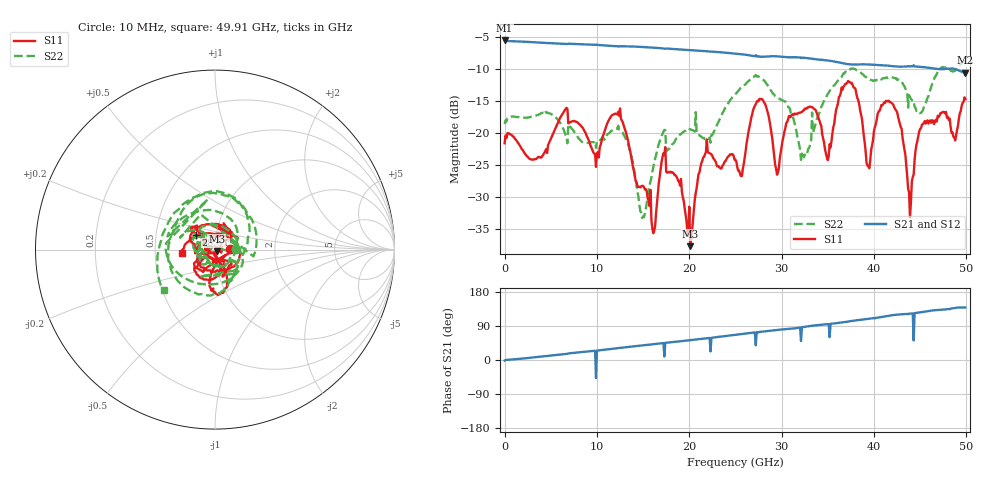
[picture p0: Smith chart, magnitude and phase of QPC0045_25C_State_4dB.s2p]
!File name = QPC0045_25C_State_4dB.s2p
!Date Time: 2024/05/02 05:42:16 AM
!Cal Ref Plane:TRL
!TEMP = 25C
!Vdd(V) = 3.15
!Vss(V) = 0.000
# GHz  S  DB  R  50
!%	Freq(GHz)  S11(dB)  S11(deg)  S21(dB)  S21(deg)  S12(dB)  S12(deg)  S22(dB)  S22(deg)
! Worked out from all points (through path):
!   500 points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, 10 MHz to 49.91 GHz, reference 50 ohm
!   highest |S21| = -5.60 dB at 10 MHz (marker M1); lowest = -10.7 dB at 49.91 GHz (marker M2)
!   lowest |S11| = -37.7 dB at 20.11 GHz (marker M3), VSWR 1.03, Z = 51 - j0.859 ohm
!   |S11| at or under -10 dB: start of sweep to end of sweep
!   |S22| runs from -33.3 to -8.8 dB; largest |S21 - S12| = 0.0015
!   S11 on the Smith chart (normalised r, x): 10 MHz: 1.18, +0.00; 28.61 GHz: 0.80, +0.14; 49.91 GHz: 0.69, -0.03
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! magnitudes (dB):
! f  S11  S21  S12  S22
! 10 MHz  -21.7  -5.6  -5.6  -18.7
! 8.41 GHz  -19.2  -6.2  -6.2  -21.5
! 10.01 GHz  -23.3  -6.3  -6.3  -21.3
! 12.51 GHz  -16.2  -6.5  -6.5  -19.5
! 15.01 GHz  -28.3  -6.6  -6.6  -33.1
! 16.11 GHz  -35.7  -6.7  -6.7  -25.4
! 16.71 GHz  -27.9  -6.8  -6.8  -21.8
! 17.21 GHz  -23.2  -6.9  -6.9  -19.8
! 20.11 GHz  -37.7  -7.1  -7.1  -19.5
! 21.71 GHz  -23.4  -7.3  -7.3  -21.0
! 25.01 GHz  -24.2  -7.7  -7.7  -14.0
! 28.61 GHz  -17.5  -8.1  -8.1  -12.9
! 29.51 GHz  -26.6  -8.1  -8.1  -14.5
! 32.31 GHz  -16.6  -8.3  -8.3  -23.6
! 33.31 GHz  -16.0  -8.4  -8.4  -16.8
! 34.91 GHz  -23.8  -8.7  -8.7  -14.2
! 37.51 GHz  -12.3  -9.3  -9.3  -10.0
! 39.41 GHz  -25.3  -9.4  -9.4  -11.5
! 41.61 GHz  -15.0  -9.6  -9.5  -11.4
! 43.91 GHz  -33.2  -9.6  -9.6  -14.5
! 45.11 GHz  -19.2  -9.7  -9.7  -16.9
! 49.91 GHz  -14.7  -10.7  -10.6  -8.8
